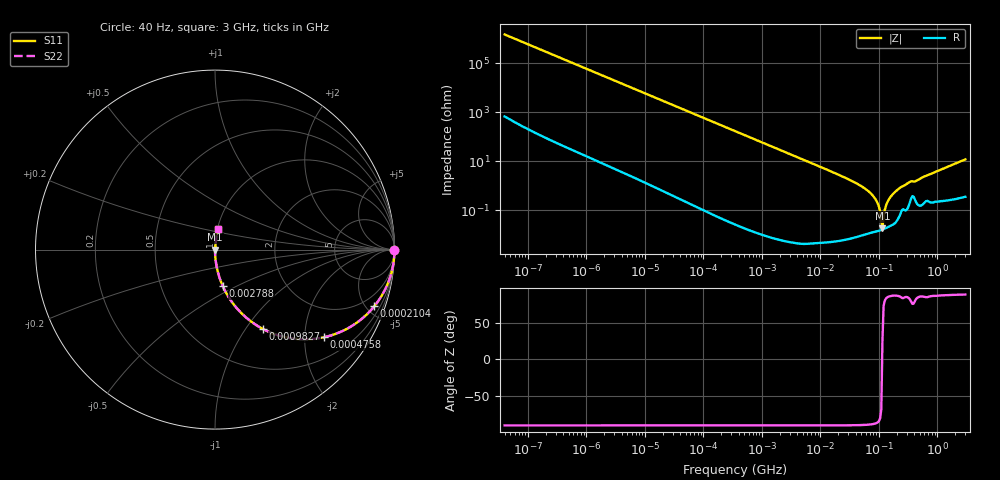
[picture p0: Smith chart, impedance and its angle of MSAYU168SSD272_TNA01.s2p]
! MSAYU168SSD272_TNA01  S-PARAMETER MODEL  ( General Type )
! Model Generated by TAIYO YUDEN Corporation (http://www.ty-top.com)
! Version 2.0
! TAIYO YUDEN Control No. 030711
! Copyright(c) 2003 TAIYO YUDEN CO.,LTD. All Rights Reserved.
! Product Description (link to TY-COMPAS)
! https://ds.yuden.co.jp/TYCOMPAS/or/detail?pn=MSAYU168SSD272KTNA01&u=M
! Products Name : Multilayer Ceramic Capacitors
! Characteristics :
!  Capacitance : 2700 pF , Rated Voltage : 50V
!  Case Size : 1.6 x 0.8 / 0.063 x 0.031 [mm/inch] , Thickness : 0.8 / 0.031 [mm/inch]
!  (Conditions: Temperature = 25 degC , DC Bias Current/Voltage = 0A / 0V)
! External Node Assignments :
!  1  o---| |---o  2
! GND o---------o GND
! Frequency Range : 40Hz  -  3GHz  [ 401 STEP ]
# MHz S RI R 50
! Freq[MHz].  S11 Real  S11 Imag  S21 Real  S21 Imag  S12 Real  S12 Imag  S22 Real  S22 Imag
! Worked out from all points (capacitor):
!   401 points, 40 Hz to 3 GHz, reference 50 ohm
!   read as one part in series: C = 2.69 nF near 44 Hz
!   lowest |Z| = 18.1 mohm at 114.7 MHz (marker M1)
!   series resonance near 113.8 MHz, so ESL is about 730 pH
!   S11 on the Smith chart (normalised r, x): 40 Hz: open; 210.4 kHz: 1.00, -5.62; 475.8 kHz: 1.00, -2.48; 982.7 kHz: 1.00, -1.20; 2.788 MHz: 1.00, -0.42; 3 GHz: 1.01, +0.24
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4e-05  1 -6.77e-05  3.5e-08 6.77e-05  3.5e-08 6.77e-05  1 -6.77e-05
6.6e-05  1 -0.000112  5.5e-08 0.000112  5.5e-08 0.000112  1 -0.000112
0.000834  1 -0.00141  2.37e-06 0.00141  2.37e-06 0.00141  1 -0.00141
0.017386  0.9991 -0.0294  0.000871 0.0294  0.000871 0.0294  0.9991 -0.0294
0.07088  0.9858 -0.1182  0.0142 0.1182  0.0142 0.1182  0.9858 -0.1182
0.210391  0.8875 -0.3159  0.1125 0.3159  0.1125 0.3159  0.8875 -0.3159
0.362475  0.7266 -0.4456  0.2734 0.4456  0.2734 0.4456  0.7266 -0.4456
0.475778  0.6068 -0.4884  0.3932 0.4884  0.3932 0.4884  0.6068 -0.4884
0.982668  0.2657 -0.4416  0.7343 0.4416  0.7343 0.4416  0.2657 -0.4416
2.78755  0.043 -0.2028  0.957 0.2028  0.957 0.2028  0.043 -0.2028
7.222098  0.00664 -0.081  0.9934 0.081  0.9934 0.081  0.00664 -0.081
60.81113  0.000155 -0.00695  0.9998 0.00695  0.9998 0.00695  0.000155 -0.00695
87.39454  0.000141 -0.00277  0.9999 0.00277  0.9999 0.00277  0.000141 -0.00277
95.68847  0.000144 -0.00183  0.9999 0.00183  0.9999 0.00183  0.000144 -0.00183
104.7695  0.000151 -0.000858  0.9998 0.000858  0.9998 0.000858  0.000151 -0.000858
114.7124  0.000162 7.93e-05  0.9998 -7.93e-05  0.9998 -7.93e-05  0.000162 7.93e-05
120.0322  0.00017 0.000552  0.9998 -0.000552  0.9998 -0.000552  0.00017 0.000552
137.5184  0.000201 0.00198  0.9998 -0.00198  0.9998 -0.00198  0.000201 0.00198
150.5692  0.000228 0.00297  0.9998 -0.00297  0.9998 -0.00297  0.000228 0.00297
206.7996  0.000447 0.00677  0.9996 -0.00677  0.9996 -0.00677  0.000447 0.00677
325.4065  0.00179 0.0135  0.9982 -0.0135  0.9982 -0.0135  0.00179 0.0135
3000  0.0172 0.1161  0.9828 -0.1161  0.9828 -0.1161  0.0172 0.1161
